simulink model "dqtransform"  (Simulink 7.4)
settings: Solver=ode45  StartTime=0.0  StopTime=1  MaxStep=1e-4  RelTol=1e-3
libraries: simulink x3

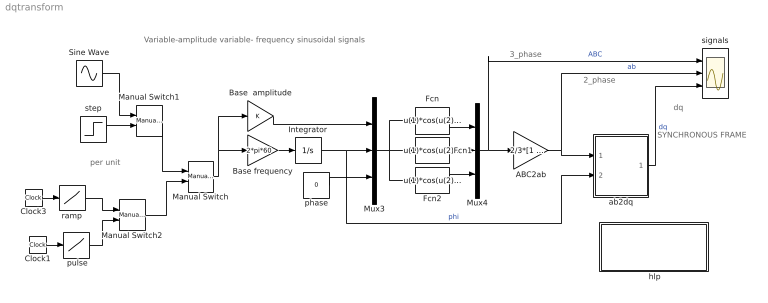
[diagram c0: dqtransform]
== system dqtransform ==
  note: Variable-amplitude variable- frequency sinusoidal signals
  note: 3_phase
  note: 2_phase
  note: dq
  note: per unit
  note: SYNCHRONOUS FRAME
  " hlp" : Subsystem
  " pulse" : Lookup  InputValues="[0  .1 .101 .8  .801 1]"  Table=[0 0 1 1 0 0]  OutDataType=sfix(16)  OutScaling=2^0
  " ramp " : Lookup  InputValues=[0 0.8 2]  Table=[0 1.0 1.0]  OutDataType=sfix(16)  OutScaling=2^0
  ABC2ab : Gain  Gain=2/3*[1 -0.5 -0.5;0 sqrt(3)/2 -sqrt(3)/2]  Multiplication=Matrix(K*u)  ParameterDataType=sfix(16)  ParameterScaling=2^0  OutDataType=sfix(16)  OutScaling=2^0
  Base frequency : Gain  Gain=2*pi*60  ParameterDataType=sfix(16)  ParameterScaling=2^0  OutDataType=sfix(16)  OutScaling=2^0
  Base  amplitude : Gain  ParameterDataType=sfix(16)  ParameterScaling=2^0  OutDataType=sfix(16)  OutScaling=2^0
  Clock1 : Clock
  Clock3 : Clock
  Fcn : Fcn  Expr=u(1)*cos(u(2)+u(3))
  Fcn1 : Fcn  Expr=u(1)*cos(u(2)-2*pi/3+u(3))
  Fcn2 : Fcn  Expr=u(1)*cos(u(2)+2*pi/3+u(3))
  Integrator : Integrator
  Manual Switch : simulink/Signal Routing/Manual Switch  SystemSampleTime=-1  sw=0  action=0  varsize=off
  Manual Switch1 : simulink/Signal Routing/Manual Switch  SystemSampleTime=-1  sw=0  action=0  varsize=off
  Manual Switch2 : simulink/Signal Routing/Manual Switch  SystemSampleTime=-1  sw=1  action=0  varsize=off
  Mux3 : Mux  Inputs=3
  Mux4 : Mux  Inputs=3
  Sine Wave : Sin  Amplitude=.2  Bias=0  Frequency=7  Phase=0  Samples=10  SampleTime=0
  ab2dq : Subsystem
  phase : Constant  Value=0  OutDataType=sfix(16)  OutScaling=2^0
  signals : Scope  NumInputPorts=3
  step : Step  Time=.2  Before=1  After=5/6  SampleTime=0
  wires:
  ab2dq/1(dq) -> signals/3  "dq"
  Mux4/1 -> ABC2ab/1, signals/1  "ABC"
  Fcn/1 -> Mux4/1
  Fcn1/1 -> Mux4/2
  Fcn2/1 -> Mux4/3
  ABC2ab/1 -> ab2dq/1(ab), signals/2  "ab"
  Base frequency/1 -> Integrator/1
  Integrator/1 -> Mux3/2, ab2dq/2(phi)  "phi"
  Mux3/1 -> Fcn1/1, Fcn/1, Fcn2/1
  Base  amplitude/1 -> Mux3/1
  phase/1 -> Mux3/3
  Clock3/1 -> " ramp "/1
  Manual Switch/1 -> Base  amplitude/1, Base frequency/1
  Sine Wave/1 -> Manual Switch1/1
  step/1 -> Manual Switch1/2
  Manual Switch1/1 -> Manual Switch/1
  Clock1/1 -> " pulse"/1
  " ramp "/1 -> Manual Switch2/1
  " pulse"/1 -> Manual Switch2/2
  Manual Switch2/1 -> Manual Switch/2

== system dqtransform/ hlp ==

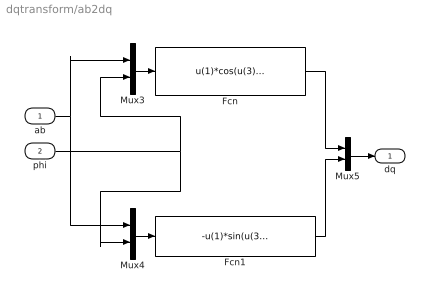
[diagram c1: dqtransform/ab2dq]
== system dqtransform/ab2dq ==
  ab : Inport  OutDataType=sfix(16)  OutScaling=2^0
  phi : Inport  Port=2  OutDataType=sfix(16)  OutScaling=2^0
  Fcn : Fcn  Expr=u(1)*cos(u(3))+u(2)*sin(u(3))
  Fcn1 : Fcn  Expr=-u(1)*sin(u(3))+u(2)*cos(u(3))
  Mux3 : Mux  Inputs=2
  Mux4 : Mux  Inputs=2
  Mux5 : Mux  Inputs=2
  dq : Outport
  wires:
  Mux3/1 -> Fcn/1
  Mux4/1 -> Fcn1/1
  ab/1 -> Mux3/1, Mux4/1
  phi/1 -> Mux3/2, Mux4/2
  Fcn1/1 -> Mux5/2
  Fcn/1 -> Mux5/1
  Mux5/1 -> dq/1
